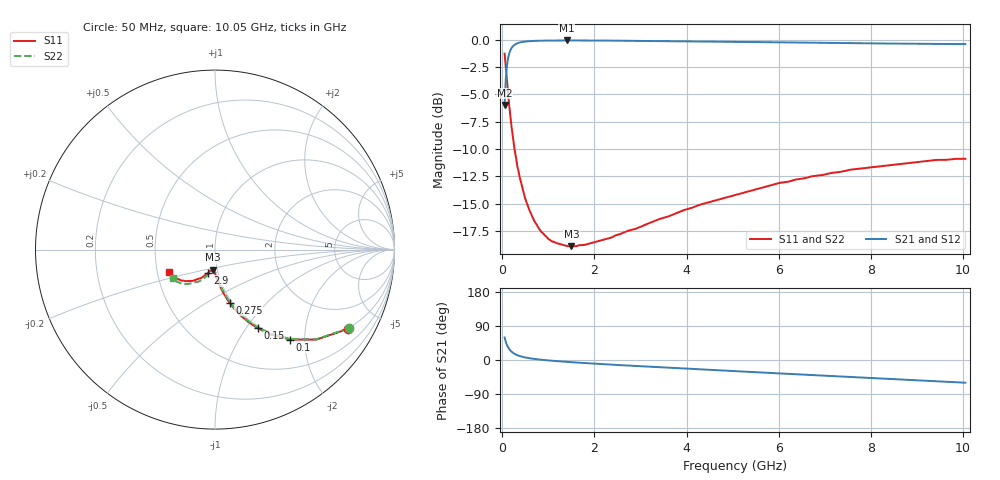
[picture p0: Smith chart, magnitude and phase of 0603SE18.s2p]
! AVX Thin Film Operation		Date: August 2001
! Description: Accu-P® Series, Thin Film, SMD, RF Capacitor
! Part Number: 06033J180FBT
! 50 MHz  -  10.05 GHz
! Serial Measurements
# mhz S db R 50
!	S11		S21		S12		S22
!	dB	Phase	dB	Phase	dB	Phase	dB	Phase
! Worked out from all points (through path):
!   401 points, 50 MHz to 10.05 GHz, reference 50 ohm
!   highest |S21| = -0.06 dB at 1.4 GHz (marker M1); lowest = -6.0 dB at 50 MHz (marker M2)
!   group delay of S21, straight-line fit = 19.3 ps
!   lowest |S11| = -18.9 dB at 1.5 GHz (marker M3), VSWR 1.26, Z = 47.5 - j10.8 ohm
!   |S11| at or under -10 dB: 265.7 MHz to end of sweep
!   |S22| runs from -18.9 to -1.3 dB; largest |S21 - S12| = 0
!   S11 on the Smith chart (normalised r, x): 50 MHz: 0.97, -3.38; 100 MHz: 0.97, -1.70; 150 MHz: 0.97, -1.14; 275 MHz: 0.97, -0.63; 2.9 GHz: 0.89, -0.24; 10.05 GHz: 0.58, -0.16
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50  -1.27 -30.7  -5.97 59.4  -5.97 59.4  -1.27 -30.5
100  -3.71 -50.2  -2.42 39.9  -2.42 39.9  -3.71 -49.9
125  -4.92 -56.6  -1.70 33.6  -1.70 33.6  -4.92 -56.2
150  -6.03 -61.4  -1.25 28.8  -1.25 28.8  -6.03 -61.0
175  -7.02 -65.2  -0.96 25.1  -0.96 25.1  -7.02 -64.7
200  -7.95 -68.2  -0.76 22.0  -0.76 22.0  -7.95 -67.7
275  -10.27 -74.6  -0.43 15.7  -0.43 15.7  -10.27 -73.9
375  -12.54 -79.8  -0.25 10.6  -0.25 10.6  -12.54 -78.8
475  -14.19 -83.1  -0.17 7.3  -0.17 7.3  -14.19 -81.8
550  -15.16 -85.0  -0.14 5.5  -0.14 5.5  -15.16 -83.5
700  -16.64 -87.9  -0.10 2.7  -0.10 2.7  -16.64 -86.2
825  -17.46 -89.9  -0.08 0.9  -0.08 0.9  -17.46 -87.8
1025  -18.31 -92.3  -0.07 -1.4  -0.07 -1.4  -18.31 -90.0
1400  -18.88 -96.0  -0.06 -5.0  -0.06 -5.0  -18.88 -93.3
1500  -18.90 -96.8  -0.06 -5.8  -0.06 -5.8  -18.90 -94.1
1725  -18.80 -98.7  -0.06 -7.6  -0.06 -7.6  -18.80 -95.8
2900  -17.30 -107.0  -0.09 -15.8  -0.09 -15.8  -17.20 -104.0
3400  -16.43 -110.8  -0.11 -19.1  -0.11 -19.1  -16.43 -106.9
5050  -14.22 -121.4  -0.18 -29.5  -0.18 -29.5  -14.12 -116.4
6725  -12.50 -132.0  -0.27 -39.7  -0.27 -39.7  -12.49 -127.0
8400  -11.49 -143.1  -0.34 -50.0  -0.34 -50.0  -11.39 -136.2
10050  -10.90 -153.6  -0.39 -60.0  -0.39 -60.0  -10.90 -145.8
